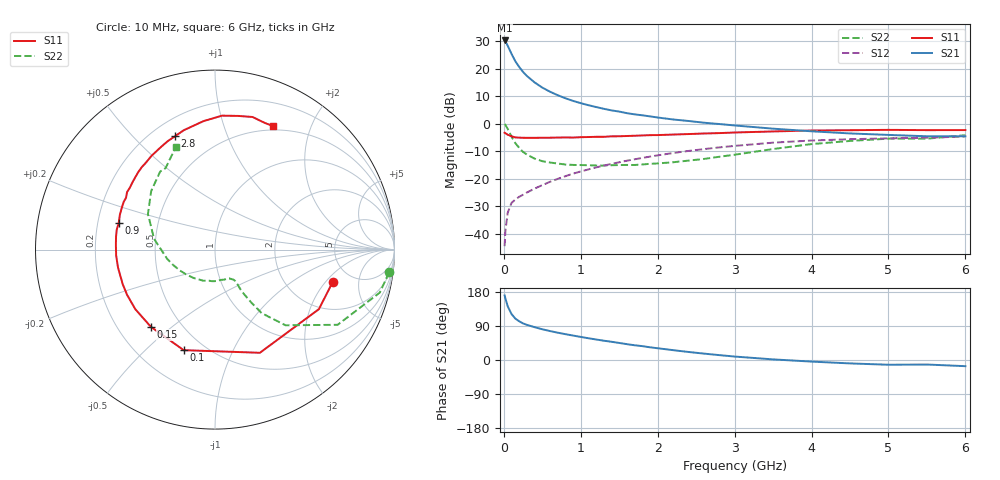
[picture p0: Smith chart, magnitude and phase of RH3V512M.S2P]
! SIEMENS Small Signal Semiconductors
! BFR106
! Si NPN RF Bipolar Junction Transistor in SOT23
! VCE = 3.5 V  IC = 12 mA
! Common Emitter S-Parameters:  August  1996
# GHz  S  MA  R  50
!  f  S11  S21  S12  S22
! GHz  MAG  ANG  MAG  ANG  MAG  ANG  MAG  ANG
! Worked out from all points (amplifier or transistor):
!   36 points, 10 MHz to 6 GHz, reference 50 ohm
!   highest |S21| = 30.2 dB at 10 MHz (marker M1)
!   |S21| within 3 dB of that: start of sweep to 68.47 MHz
!   unconditionally stable (mu >= 1): 455.7 MHz to 2.126 GHz; 5.218 GHz to end of sweep
!   at 250 MHz: K = 0.77, MSG = 22.3 dB, |S12| = -25.9 dB
!   at 1.4 GHz: K = 1.09, MAG = 7.9 dB, |S12| = -14.7 dB
!   at 6 GHz: K = 1.01, MAG = -0.5 dB, |S12| = -4.7 dB
!   S11 on the Smith chart (normalised r, x): 10 MHz: 3.57, -2.39; 100 MHz: 0.39, -0.66; 150 MHz: 0.34, -0.42; 900 MHz: 0.29, +0.12; 2.8 GHz: 0.29, +0.67; 6 GHz: 0.45, +1.48
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0.01  0.6803 -15.3  32.38 170.4  0.0059 85.9  0.9786 -7.4
0.02  0.6673 -29.8  31.32 162.7  0.0111 77.1  0.9491 -14.6
0.05  0.6269 -66.5  26.04 141.8  0.0239 63.1  0.8018 -31.5
0.1  0.5868 -107.3  18.45 121.3  0.0361 51.1  0.5767 -47.0
0.15  0.5592 -129.7  13.53 109.1  0.0416 47.4  0.4395 -53.7
0.2  0.5544 -143.2  10.67 102.1  0.0467 48.2  0.3602 -55.5
0.25  0.5509 -152.8  8.664 96.5  0.0508 49.7  0.3043 -56.7
0.3  0.5491 -159.5  7.314 92.7  0.0558 51.9  0.2732 -57.4
0.4  0.5495 -169.4  5.592 86.6  0.0657 54.9  0.2301 -57.1
0.5  0.5517 -176.5  4.503 81.1  0.076 57.9  0.2069 -57.3
0.6  0.5528 177.5  3.789 76.4  0.0872 59.7  0.1956 -58.6
0.7  0.5561 172.5  3.276 72.1  0.0986 61.2  0.1876 -60.9
0.9  0.5566 164.5  2.58 64.5  0.1228 62.2  0.1769 -65.5
1.1  0.5687 156.2  2.155 57.4  0.1468 62.1  0.1747 -73.5
1.3  0.5739 149.7  1.853 50.9  0.1723 61.3  0.1725 -81.2
1.6  0.5936 140.6  1.543 41.8  0.2111 59.1  0.1768 -95.6
2.2  0.6308 124.1  1.186 26.0  0.2913 52.5  0.1979 -126.8
2.8  0.6698 109.4  0.98 12.9  0.3682 43.8  0.2489 -160.0
3.5  0.7184 95.2  0.807 1.6  0.4492 32.6  0.3443 170.1
4.5  0.7562 80.0  0.661 -9.0  0.519 15.9  0.4828 137.4
5.5  0.7583 68.5  0.587 -11.9  0.5523 5.2  0.5311 121.2
6  0.7605 64.8  0.586 -16.3  0.5815 -2.5  0.6131 110.8
